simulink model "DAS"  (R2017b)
settings: Solver=FixedStepDiscrete  StartTime=0.0  StopTime=10.0  FixedStep=0.01  RelTol=1e-3  EnableMultiTasking=on
undefined symbols (not defined in the file): CcDAS_ACModeCurtLim_A, CcDAS_ACModeCurtTiLim_ms, CcDAS_BMSOperationConfirmTi_ms, CcDAS_CellMaxTempLim1_C, CcDAS_CellMaxTempLim2_C, CcDAS_CellMaxTempLim3_C, CcDAS_CellMaxTempLim4_C, CcDAS_CellMinTempHiLim_C, CcDAS_CellMinTempLowLim_C, CcDAS_CellMinTempMidLim_C, CcDAS_CellTempDiffLim_C, CcDAS_DCModeCurtTiLim_ms, CcDAS_HVSafetyNVMStoreTi_ms, CcDAS_OCVSOCDiffLim1_numb, CcDAS_OCVSOCDiffLim2_numb, CcDAS_PackCurrLim_A, CcDAS_SOCHighLim_numb, CcDAS_SOCLowerLim_numb, CcDAS_SOHLowerLim_numb, CcDAS_SOHLowerLimSale_numb, DAS_MIN2MS_NUMB, DAS_RUNTIME100_MS, DAS_RUNTIME10_MS, DAS_STATSTIMEMAX_MIN, DAS_STATSTIMEMIN_MIN, DAS_STATSTIMESMAX_NUMB, DAS_STATSTIMESMIN_NUMB, DAS_TIMESONE_NUMB, Enum_CTCCtrCtlConnMode
libraries: AIWAYS_Powertrain_BMS_lib x268
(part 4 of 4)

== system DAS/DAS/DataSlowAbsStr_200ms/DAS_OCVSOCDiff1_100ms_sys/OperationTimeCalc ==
  Enable : EnablePort
  Constant1 : Constant  Value=DAS_MIN2MS_NUMB
  Constant10 : Constant  Value=DAS_RUNTIME100_MS
  Constant2 : Constant  Value=DAS_STATSTIMEMIN_MIN
  Constant3 : Constant  Value=DAS_STATSTIMEMAX_MIN
  Data Store Read : AIWAYS_Powertrain_BMS_lib/Signals/Data Store Read  Priority=0  DSR=EcNVM_OCVSOCDiffTi1_min
  Data Store Write : AIWAYS_Powertrain_BMS_lib/Signals/Data Store Write  DSW=EcNVM_OCVSOCDiffTi1_min
  Data Type Conversion : DataTypeConversion  OutDataTypeStr=single
  Data Type Conversion1 : DataTypeConversion  OutDataTypeStr=single
  Limiter : AIWAYS_Powertrain_BMS_lib/Nonlinear Blocks/Limiter
  OverWrite : AIWAYS_Powertrain_BMS_lib/Signals/OverWrite  OverWrite_Value=CcDAS_OCVSOCDiffTi1Ovr_min  OverWrite_flag=CbDAS_OCVSOCDiffTi1OvrSwt_flg
  Product1 : Product  Inputs=*/  OutDataTypeStr=Inherit: Inherit via back propagation
  Sum : Sum  OutDataTypeStr=Inherit: Inherit via back propagation  RndMeth=Zero
  GcDAS_OCVSOCDiffTi1_min : Outport
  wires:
  Data Store Read/1 -> Sum/1
  Constant10/1 -> Data Type Conversion/1
  Data Type Conversion/1 -> Product1/1
  Product1/1 -> Sum/2
  Constant1/1 -> Data Type Conversion1/1
  Data Type Conversion1/1 -> Product1/2
  Sum/1 -> Limiter/3
  Limiter/1 -> OverWrite/1
  Constant2/1 -> Limiter/2
  Constant3/1 -> Limiter/1
  OverWrite/1 -> Data Store Write/1, GcDAS_OCVSOCDiffTi1_min/1  "GcDAS_OCVSOCDiffTi1_min"

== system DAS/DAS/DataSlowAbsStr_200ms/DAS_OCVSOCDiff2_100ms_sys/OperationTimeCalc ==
  Enable : EnablePort
  Constant1 : Constant  Value=DAS_MIN2MS_NUMB
  Constant10 : Constant  Value=DAS_RUNTIME100_MS
  Constant2 : Constant  Value=DAS_STATSTIMEMIN_MIN
  Constant3 : Constant  Value=DAS_STATSTIMEMAX_MIN
  Data Store Read : AIWAYS_Powertrain_BMS_lib/Signals/Data Store Read  Priority=0  DSR=EcNVM_OCVSOCDiffTi2_min
  Data Store Write : AIWAYS_Powertrain_BMS_lib/Signals/Data Store Write  DSW=EcNVM_OCVSOCDiffTi2_min
  Data Type Conversion : DataTypeConversion  OutDataTypeStr=single
  Data Type Conversion1 : DataTypeConversion  OutDataTypeStr=single
  Limiter : AIWAYS_Powertrain_BMS_lib/Nonlinear Blocks/Limiter
  OverWrite : AIWAYS_Powertrain_BMS_lib/Signals/OverWrite  OverWrite_Value=CcDAS_OCVSOCDiffTi2Ovr_min  OverWrite_flag=CbDAS_OCVSOCDiffTi2OvrSwt_flg
  Product1 : Product  Inputs=*/  OutDataTypeStr=Inherit: Inherit via back propagation
  Sum : Sum  OutDataTypeStr=Inherit: Inherit via back propagation  RndMeth=Zero
  GcDAS_OCVSOCDiffTi2_min : Outport
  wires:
  Data Store Read/1 -> Sum/1
  Constant10/1 -> Data Type Conversion/1
  Data Type Conversion/1 -> Product1/1
  Product1/1 -> Sum/2
  Constant1/1 -> Data Type Conversion1/1
  Data Type Conversion1/1 -> Product1/2
  Sum/1 -> Limiter/3
  Limiter/1 -> OverWrite/1
  Constant2/1 -> Limiter/2
  Constant3/1 -> Limiter/1
  OverWrite/1 -> Data Store Write/1, GcDAS_OCVSOCDiffTi2_min/1  "GcDAS_OCVSOCDiffTi2_min"

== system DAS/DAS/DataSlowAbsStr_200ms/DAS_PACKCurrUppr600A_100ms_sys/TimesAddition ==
  Enable : EnablePort
  ACC_GbACC_ACChrgMismatch_flg : AIWAYS_Powertrain_BMS_lib/Signals/OverWrite  OverWrite_Value=CcDAS_TFPackCrntSafCntOvr_numb  OverWrite_flag=CbDAS_TFPackCrntSafCntOvrSwt_flg
  Constant : Constant  Value=DAS_TIMESONE_NUMB
  Constant4 : Constant  Value=DAS_STATSTIMESMIN_NUMB
  Constant5 : Constant  Value=DAS_STATSTIMESMAX_NUMB
  Data Store Read : AIWAYS_Powertrain_BMS_lib/Signals/Data Store Read  Priority=0  DSR=EcNVM_TFPackCrntSafCnt_numb
  Data Store Write : AIWAYS_Powertrain_BMS_lib/Signals/Data Store Write  DSW=EcNVM_TFPackCrntSafCnt_numb
  Limiter : AIWAYS_Powertrain_BMS_lib/Nonlinear Blocks/Limiter
  Sum : Sum  OutDataTypeStr=Inherit: Inherit via back propagation  RndMeth=Zero
  GcDAS_TFPackCrntSafCnt_numb : Outport
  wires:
  Data Store Read/1 -> Sum/1
  Sum/1 -> Limiter/3
  ACC_GbACC_ACChrgMismatch_flg/1 -> GcDAS_TFPackCrntSafCnt_numb/1, Data Store Write/1  "GcDAS_TFPackCrntSafCnt_numb"
  Constant/1 -> Sum/2
  Constant5/1 -> Limiter/1
  Constant4/1 -> Limiter/2
  Limiter/1 -> ACC_GbACC_ACChrgMismatch_flg/1

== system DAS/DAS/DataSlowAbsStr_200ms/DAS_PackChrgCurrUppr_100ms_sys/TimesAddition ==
  Enable : EnablePort
  ACC_GbACC_ACChrgMismatch_flg : AIWAYS_Powertrain_BMS_lib/Signals/OverWrite  OverWrite_Value=CcDAS_PackChrgCurrUpprLimCntOvr_numb  OverWrite_flag=CbDAS_PackChrgCurrUpprLimCntOvrSwt_flg
  Constant : Constant  Value=DAS_TIMESONE_NUMB
  Constant4 : Constant  Value=DAS_STATSTIMESMIN_NUMB
  Constant5 : Constant  Value=DAS_STATSTIMESMAX_NUMB
  Data Store Read : AIWAYS_Powertrain_BMS_lib/Signals/Data Store Read  Priority=0  DSR=EcNVM_PackChrgCurrUpprLimCnt_numb
  Data Store Write : AIWAYS_Powertrain_BMS_lib/Signals/Data Store Write  DSW=EcNVM_PackChrgCurrUpprLimCnt_numb
  Limiter : AIWAYS_Powertrain_BMS_lib/Nonlinear Blocks/Limiter
  Sum : Sum  OutDataTypeStr=Inherit: Inherit via back propagation  RndMeth=Zero
  GcDAS_PackChrgCurrUpprLimCnt_numb : Outport
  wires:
  Data Store Read/1 -> Sum/1
  Sum/1 -> Limiter/3
  ACC_GbACC_ACChrgMismatch_flg/1 -> GcDAS_PackChrgCurrUpprLimCnt_numb/1, Data Store Write/1  "GcDAS_PackChrgCurrUpprLimCnt_numb"
  Constant/1 -> Sum/2
  Constant5/1 -> Limiter/1
  Constant4/1 -> Limiter/2
  Limiter/1 -> ACC_GbACC_ACChrgMismatch_flg/1

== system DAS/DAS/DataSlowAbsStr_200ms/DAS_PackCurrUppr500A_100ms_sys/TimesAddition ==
  Enable : EnablePort
  ACC_GbACC_ACChrgMismatch_flg : AIWAYS_Powertrain_BMS_lib/Signals/OverWrite  OverWrite_Value=CcDAS_PackCurrLim500ACntOvr_numb  OverWrite_flag=CbDAS_PackCurrLim500ACntOvrSwt_flg
  Constant : Constant  Value=DAS_TIMESONE_NUMB  OutDataTypeStr=single
  Constant4 : Constant  Value=DAS_STATSTIMEMIN_MIN  OutDataTypeStr=single
  Constant5 : Constant  Value=DAS_STATSTIMEMAX_MIN  OutDataTypeStr=single
  Data Store Read : AIWAYS_Powertrain_BMS_lib/Signals/Data Store Read  Priority=0  DSR=EcNVM_PackCurrLim500ACnt_numb
  Data Store Write : AIWAYS_Powertrain_BMS_lib/Signals/Data Store Write  DSW=EcNVM_PackCurrLim500ACnt_numb
  Data Type Conversion : DataTypeConversion  OutDataTypeStr=uint32
  Data Type Conversion1 : DataTypeConversion  OutDataTypeStr=uint32
  Data Type Conversion2 : DataTypeConversion  OutDataTypeStr=uint32
  Limiter : AIWAYS_Powertrain_BMS_lib/Nonlinear Blocks/Limiter
  Sum : Sum  OutDataTypeStr=Inherit: Inherit via back propagation  RndMeth=Zero
  GcDAS_PackCurrLim500ACnt_numb : Outport
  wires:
  Data Store Read/1 -> Sum/1
  Sum/1 -> Limiter/3
  ACC_GbACC_ACChrgMismatch_flg/1 -> GcDAS_PackCurrLim500ACnt_numb/1, Data Store Write/1  "GcDAS_PackCurrLim500ACnt_numb"
  Constant/1 -> Data Type Conversion/1
  Constant5/1 -> Data Type Conversion2/1
  Constant4/1 -> Data Type Conversion1/1
  Limiter/1 -> ACC_GbACC_ACChrgMismatch_flg/1
  Data Type Conversion/1 -> Sum/2
  Data Type Conversion1/1 -> Limiter/2
  Data Type Conversion2/1 -> Limiter/1

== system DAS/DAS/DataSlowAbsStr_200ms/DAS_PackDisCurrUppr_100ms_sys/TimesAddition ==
  Enable : EnablePort
  ACC_GbACC_ACChrgMismatch_flg : AIWAYS_Powertrain_BMS_lib/Signals/OverWrite  OverWrite_Value=CcDAS_PackDisCurrUpprLimCntOvr_numb  OverWrite_flag=CbDAS_PackDisCurrUpprLimCntOvrSwt_flg
  Constant : Constant  Value=DAS_TIMESONE_NUMB
  Constant4 : Constant  Value=DAS_STATSTIMESMIN_NUMB
  Constant5 : Constant  Value=DAS_STATSTIMESMAX_NUMB
  Data Store Read : AIWAYS_Powertrain_BMS_lib/Signals/Data Store Read  Priority=0  DSR=EcNVM_PackDisCurrUpprLimCnt_numb
  Data Store Write : AIWAYS_Powertrain_BMS_lib/Signals/Data Store Write  DSW=EcNVM_PackDisCurrUpprLimCnt_numb
  Limiter : AIWAYS_Powertrain_BMS_lib/Nonlinear Blocks/Limiter
  Sum : Sum  OutDataTypeStr=Inherit: Inherit via back propagation  RndMeth=Zero
  GcDAS_PackDisCurrUpprLimCnt_numb : Outport
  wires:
  Data Store Read/1 -> Sum/1
  Sum/1 -> Limiter/3
  ACC_GbACC_ACChrgMismatch_flg/1 -> GcDAS_PackDisCurrUpprLimCnt_numb/1, Data Store Write/1  "GcDAS_PackDisCurrUpprLimCnt_numb"
  Constant/1 -> Sum/2
  Constant5/1 -> Limiter/1
  Constant4/1 -> Limiter/2
  Limiter/1 -> ACC_GbACC_ACChrgMismatch_flg/1

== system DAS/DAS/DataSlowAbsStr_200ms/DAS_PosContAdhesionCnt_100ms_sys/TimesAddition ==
  Enable : EnablePort
  ACC_GbACC_ACChrgMismatch_flg : AIWAYS_Powertrain_BMS_lib/Signals/OverWrite  OverWrite_Value=CcDAS_PosContAdhesionCntOvr_numb  OverWrite_flag=CbDAS_PosContAdhesionCntOvrSwt_flg
  Constant : Constant  Value=DAS_TIMESONE_NUMB
  Constant4 : Constant  Value=DAS_STATSTIMESMIN_NUMB
  Constant5 : Constant  Value=DAS_STATSTIMESMAX_NUMB
  Data Store Read : AIWAYS_Powertrain_BMS_lib/Signals/Data Store Read  Priority=0  DSR=EcNVM_PosContAdhesionCnt_numb
  Data Store Write : AIWAYS_Powertrain_BMS_lib/Signals/Data Store Write  DSW=EcNVM_PosContAdhesionCnt_numb
  Limiter : AIWAYS_Powertrain_BMS_lib/Nonlinear Blocks/Limiter
  Sum : Sum  OutDataTypeStr=Inherit: Inherit via back propagation  RndMeth=Zero
  GcDAS_PosContAdhesionCnt_numb : Outport
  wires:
  Data Store Read/1 -> Sum/1
  Sum/1 -> Limiter/3
  ACC_GbACC_ACChrgMismatch_flg/1 -> GcDAS_PosContAdhesionCnt_numb/1, Data Store Write/1  "GcDAS_PosContAdhesionCnt_numb"
  Constant/1 -> Sum/2
  Constant5/1 -> Limiter/1
  Constant4/1 -> Limiter/2
  Limiter/1 -> ACC_GbACC_ACChrgMismatch_flg/1

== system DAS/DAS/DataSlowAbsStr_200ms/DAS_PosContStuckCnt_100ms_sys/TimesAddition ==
  Enable : EnablePort
  ACC_GbACC_ACChrgMismatch_flg : AIWAYS_Powertrain_BMS_lib/Signals/OverWrite  OverWrite_Value=CcDAS_PosContStuckCntOvr_numb  OverWrite_flag=CbDAS_PosContStuckCntOvrSwt_flg
  Constant : Constant  Value=DAS_TIMESONE_NUMB
  Constant4 : Constant  Value=DAS_STATSTIMESMIN_NUMB
  Constant5 : Constant  Value=DAS_STATSTIMESMAX_NUMB
  Data Store Read : AIWAYS_Powertrain_BMS_lib/Signals/Data Store Read  Priority=0  DSR=EcNVM_PosContStuckCnt_numb
  Data Store Write : AIWAYS_Powertrain_BMS_lib/Signals/Data Store Write  DSW=EcNVM_PosContStuckCnt_numb
  Limiter : AIWAYS_Powertrain_BMS_lib/Nonlinear Blocks/Limiter
  Sum : Sum  OutDataTypeStr=Inherit: Inherit via back propagation  RndMeth=Zero
  GcDAS_PosContStuckCnt_numb : Outport
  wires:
  Data Store Read/1 -> Sum/1
  Sum/1 -> Limiter/3
  ACC_GbACC_ACChrgMismatch_flg/1 -> GcDAS_PosContStuckCnt_numb/1, Data Store Write/1  "GcDAS_PosContStuckCnt_numb"
  Constant/1 -> Sum/2
  Constant5/1 -> Limiter/1
  Constant4/1 -> Limiter/2
  Limiter/1 -> ACC_GbACC_ACChrgMismatch_flg/1

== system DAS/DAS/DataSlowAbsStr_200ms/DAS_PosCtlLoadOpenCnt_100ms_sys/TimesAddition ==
  Enable : EnablePort
  ACC_GbACC_ACChrgMismatch_flg : AIWAYS_Powertrain_BMS_lib/Signals/OverWrite  OverWrite_Value=CcDAS_PosCtlLoadOpenCntOvr_numb  OverWrite_flag=CbDAS_PosCtlLoadOpenCntOvrSwt_flg
  Constant : Constant  Value=DAS_TIMESONE_NUMB
  Constant4 : Constant  Value=DAS_STATSTIMESMIN_NUMB
  Constant5 : Constant  Value=DAS_STATSTIMESMAX_NUMB
  Data Store Read : AIWAYS_Powertrain_BMS_lib/Signals/Data Store Read  Priority=0  DSR=EcNVM_PosCtlLoadOpenCnt_numb
  Data Store Write : AIWAYS_Powertrain_BMS_lib/Signals/Data Store Write  DSW=EcNVM_PosCtlLoadOpenCnt_numb
  Limiter : AIWAYS_Powertrain_BMS_lib/Nonlinear Blocks/Limiter
  Sum : Sum  OutDataTypeStr=Inherit: Inherit via back propagation  RndMeth=Zero
  GcDAS_PosCtlLoadOpenCnt_numb : Outport
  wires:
  Data Store Read/1 -> Sum/1
  Sum/1 -> Limiter/3
  ACC_GbACC_ACChrgMismatch_flg/1 -> GcDAS_PosCtlLoadOpenCnt_numb/1, Data Store Write/1  "GcDAS_PosCtlLoadOpenCnt_numb"
  Constant/1 -> Sum/2
  Constant5/1 -> Limiter/1
  Constant4/1 -> Limiter/2
  Limiter/1 -> ACC_GbACC_ACChrgMismatch_flg/1

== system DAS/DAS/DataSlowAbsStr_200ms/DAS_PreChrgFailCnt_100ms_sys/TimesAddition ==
  Enable : EnablePort
  ACC_GbACC_ACChrgMismatch_flg : AIWAYS_Powertrain_BMS_lib/Signals/OverWrite  OverWrite_Value=CcDAS_PreChrgFailCntOvr_numb  OverWrite_flag=CbDAS_PreChrgFailCntOvrSwt_flg
  Constant : Constant  Value=DAS_TIMESONE_NUMB
  Constant4 : Constant  Value=DAS_STATSTIMESMIN_NUMB
  Constant5 : Constant  Value=DAS_STATSTIMESMAX_NUMB
  Data Store Read : AIWAYS_Powertrain_BMS_lib/Signals/Data Store Read  Priority=0  DSR=EcNVM_PreChrgFailCnt_numb
  Data Store Write : AIWAYS_Powertrain_BMS_lib/Signals/Data Store Write  DSW=EcNVM_PreChrgFailCnt_numb
  Limiter : AIWAYS_Powertrain_BMS_lib/Nonlinear Blocks/Limiter
  Sum : Sum  OutDataTypeStr=Inherit: Inherit via back propagation  RndMeth=Zero
  GcDAS_PreChrgFailCnt_numb : Outport
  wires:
  Data Store Read/1 -> Sum/1
  Sum/1 -> Limiter/3
  ACC_GbACC_ACChrgMismatch_flg/1 -> GcDAS_PreChrgFailCnt_numb/1, Data Store Write/1  "GcDAS_PreChrgFailCnt_numb"
  Constant/1 -> Sum/2
  Constant5/1 -> Limiter/1
  Constant4/1 -> Limiter/2
  Limiter/1 -> ACC_GbACC_ACChrgMismatch_flg/1

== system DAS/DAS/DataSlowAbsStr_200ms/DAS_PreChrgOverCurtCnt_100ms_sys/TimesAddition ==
  Enable : EnablePort
  ACC_GbACC_ACChrgMismatch_flg : AIWAYS_Powertrain_BMS_lib/Signals/OverWrite  OverWrite_Value=CcDAS_PreChrgOvrCurrCntOvr_numb  OverWrite_flag=CbDAS_PreChrgOvrCurrCntOvrSwt_flg
  Constant : Constant  Value=DAS_TIMESONE_NUMB
  Constant4 : Constant  Value=DAS_STATSTIMESMIN_NUMB
  Constant5 : Constant  Value=DAS_STATSTIMESMAX_NUMB
  Data Store Read : AIWAYS_Powertrain_BMS_lib/Signals/Data Store Read  Priority=0  DSR=EcNVM_PreChrgOvrCurrCnt_numb
  Data Store Write : AIWAYS_Powertrain_BMS_lib/Signals/Data Store Write  DSW=EcNVM_PreChrgOvrCurrCnt_numb
  Limiter : AIWAYS_Powertrain_BMS_lib/Nonlinear Blocks/Limiter
  Sum : Sum  OutDataTypeStr=Inherit: Inherit via back propagation  RndMeth=Zero
  GcDAS_PreChrgOvrCurrCnt_numb : Outport
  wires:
  Data Store Read/1 -> Sum/1
  Sum/1 -> Limiter/3
  ACC_GbACC_ACChrgMismatch_flg/1 -> GcDAS_PreChrgOvrCurrCnt_numb/1, Data Store Write/1  "GcDAS_PreChrgOvrCurrCnt_numb"
  Constant/1 -> Sum/2
  Constant5/1 -> Limiter/1
  Constant4/1 -> Limiter/2
  Limiter/1 -> ACC_GbACC_ACChrgMismatch_flg/1

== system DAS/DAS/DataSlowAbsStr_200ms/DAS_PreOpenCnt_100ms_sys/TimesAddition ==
  Enable : EnablePort
  ACC_GbACC_ACChrgMismatch_flg : AIWAYS_Powertrain_BMS_lib/Signals/OverWrite  OverWrite_Value=CcDAS_PreChrgOpenCntOvr_numb  OverWrite_flag=CbDAS_PreChrgOpenCntOvrSwt_flg
  Constant : Constant  Value=DAS_TIMESONE_NUMB
  Constant4 : Constant  Value=DAS_STATSTIMESMIN_NUMB
  Constant5 : Constant  Value=DAS_STATSTIMESMAX_NUMB
  Data Store Read : AIWAYS_Powertrain_BMS_lib/Signals/Data Store Read  Priority=0  DSR=EcNVM_PreChrgOpenCnt_numb
  Data Store Write : AIWAYS_Powertrain_BMS_lib/Signals/Data Store Write  DSW=EcNVM_PreChrgOpenCnt_numb
  Limiter : AIWAYS_Powertrain_BMS_lib/Nonlinear Blocks/Limiter
  Sum : Sum  OutDataTypeStr=Inherit: Inherit via back propagation  RndMeth=Zero
  GcDAS_PreChrgOpenCnt_numb : Outport
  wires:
  Data Store Read/1 -> Sum/1
  Sum/1 -> Limiter/3
  ACC_GbACC_ACChrgMismatch_flg/1 -> GcDAS_PreChrgOpenCnt_numb/1, Data Store Write/1  "GcDAS_PreChrgOpenCnt_numb"
  Constant/1 -> Sum/2
  Constant5/1 -> Limiter/1
  Constant4/1 -> Limiter/2
  Limiter/1 -> ACC_GbACC_ACChrgMismatch_flg/1

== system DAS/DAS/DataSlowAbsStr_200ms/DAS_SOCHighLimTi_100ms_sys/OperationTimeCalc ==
  Enable : EnablePort
  Constant1 : Constant  Value=DAS_MIN2MS_NUMB
  Constant10 : Constant  Value=DAS_RUNTIME100_MS
  Constant2 : Constant  Value=DAS_STATSTIMEMIN_MIN
  Constant3 : Constant  Value=DAS_STATSTIMEMAX_MIN
  Data Store Read : AIWAYS_Powertrain_BMS_lib/Signals/Data Store Read  Priority=0  DSR=EcNVM_SOCHighLimTi_min
  Data Store Write : AIWAYS_Powertrain_BMS_lib/Signals/Data Store Write  DSW=EcNVM_SOCHighLimTi_min
  Data Type Conversion : DataTypeConversion  OutDataTypeStr=single
  Data Type Conversion1 : DataTypeConversion  OutDataTypeStr=single
  Limiter : AIWAYS_Powertrain_BMS_lib/Nonlinear Blocks/Limiter
  OverWrite : AIWAYS_Powertrain_BMS_lib/Signals/OverWrite  OverWrite_Value=CcDAS_SOCHighLimTiOvr_min  OverWrite_flag=CbDAS_SOCHighLimTiOvrSwt_flg
  Product1 : Product  Inputs=*/  OutDataTypeStr=Inherit: Inherit via back propagation
  Sum : Sum  OutDataTypeStr=Inherit: Inherit via back propagation  RndMeth=Zero
  GcDAS_SOCHighLimTi_min : Outport
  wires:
  Data Store Read/1 -> Sum/1
  Constant10/1 -> Data Type Conversion/1
  Data Type Conversion/1 -> Product1/1
  Product1/1 -> Sum/2
  Constant1/1 -> Data Type Conversion1/1
  Data Type Conversion1/1 -> Product1/2
  Sum/1 -> Limiter/3
  Limiter/1 -> OverWrite/1
  Constant2/1 -> Limiter/2
  Constant3/1 -> Limiter/1
  OverWrite/1 -> Data Store Write/1, GcDAS_SOCHighLimTi_min/1  "GcDAS_SOCHighLimTi_min"

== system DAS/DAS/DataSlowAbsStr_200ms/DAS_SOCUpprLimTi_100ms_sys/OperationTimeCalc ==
  Enable : EnablePort
  Constant1 : Constant  Value=DAS_MIN2MS_NUMB
  Constant10 : Constant  Value=DAS_RUNTIME100_MS
  Constant2 : Constant  Value=DAS_STATSTIMEMIN_MIN
  Constant3 : Constant  Value=DAS_STATSTIMEMAX_MIN
  Data Store Read : AIWAYS_Powertrain_BMS_lib/Signals/Data Store Read  Priority=0  DSR=EcNVM_SOCLowLimTi_min
  Data Store Write : AIWAYS_Powertrain_BMS_lib/Signals/Data Store Write  DSW=EcNVM_SOCLowLimTi_min
  Data Type Conversion : DataTypeConversion  OutDataTypeStr=single
  Data Type Conversion1 : DataTypeConversion  OutDataTypeStr=single
  Limiter : AIWAYS_Powertrain_BMS_lib/Nonlinear Blocks/Limiter
  OverWrite : AIWAYS_Powertrain_BMS_lib/Signals/OverWrite  OverWrite_Value=CcDAS_SOCLowLimTiOvr_min  OverWrite_flag=CbDAS_SOCLowLimTiOvrSwt_flg
  Product1 : Product  Inputs=*/  OutDataTypeStr=Inherit: Inherit via back propagation
  Sum : Sum  OutDataTypeStr=Inherit: Inherit via back propagation  RndMeth=Zero
  GcDAS_SOCLowLimTi_min : Outport
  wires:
  Data Store Read/1 -> Sum/1
  Constant10/1 -> Data Type Conversion/1
  Data Type Conversion/1 -> Product1/1
  Product1/1 -> Sum/2
  Constant1/1 -> Data Type Conversion1/1
  Data Type Conversion1/1 -> Product1/2
  Sum/1 -> Limiter/3
  Limiter/1 -> OverWrite/1
  Constant2/1 -> Limiter/2
  Constant3/1 -> Limiter/1
  OverWrite/1 -> Data Store Write/1, GcDAS_SOCLowLimTi_min/1  "GcDAS_SOCLowLimTi_min"

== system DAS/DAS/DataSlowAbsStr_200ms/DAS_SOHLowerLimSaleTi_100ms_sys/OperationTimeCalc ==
  Enable : EnablePort
  Constant1 : Constant  Value=DAS_MIN2MS_NUMB
  Constant10 : Constant  Value=DAS_RUNTIME100_MS
  Constant2 : Constant  Value=DAS_STATSTIMEMIN_MIN
  Constant3 : Constant  Value=DAS_STATSTIMEMAX_MIN
  Data Store Read : AIWAYS_Powertrain_BMS_lib/Signals/Data Store Read  Priority=0  DSR=EcNVM_SOHLowerLimSaleTi_min
  Data Store Write : AIWAYS_Powertrain_BMS_lib/Signals/Data Store Write  DSW=EcNVM_SOHLowerLimSaleTi_min
  Data Type Conversion : DataTypeConversion  OutDataTypeStr=single
  Data Type Conversion1 : DataTypeConversion  OutDataTypeStr=single
  Limiter : AIWAYS_Powertrain_BMS_lib/Nonlinear Blocks/Limiter
  OverWrite : AIWAYS_Powertrain_BMS_lib/Signals/OverWrite  OverWrite_Value=CcDAS_SOHLowerLimSaleTiOvr_min  OverWrite_flag=CbDAS_SOHLowerLimSaleTiOvrSwt_flg
  Product1 : Product  Inputs=*/  OutDataTypeStr=Inherit: Inherit via back propagation
  Sum : Sum  OutDataTypeStr=Inherit: Inherit via back propagation  RndMeth=Zero
  GcDAS_SOHLowerLimSaleTi_min : Outport
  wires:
  Data Store Read/1 -> Sum/1
  Constant10/1 -> Data Type Conversion/1
  Data Type Conversion/1 -> Product1/1
  Product1/1 -> Sum/2
  Constant1/1 -> Data Type Conversion1/1
  Data Type Conversion1/1 -> Product1/2
  Sum/1 -> Limiter/3
  Limiter/1 -> OverWrite/1
  Constant2/1 -> Limiter/2
  Constant3/1 -> Limiter/1
  OverWrite/1 -> Data Store Write/1, GcDAS_SOHLowerLimSaleTi_min/1  "GcDAS_SOHLowerLimSaleTi_min"

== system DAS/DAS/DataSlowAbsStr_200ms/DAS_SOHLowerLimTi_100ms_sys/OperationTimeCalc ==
  Enable : EnablePort
  Constant1 : Constant  Value=DAS_MIN2MS_NUMB
  Constant10 : Constant  Value=DAS_RUNTIME100_MS
  Constant2 : Constant  Value=DAS_STATSTIMEMIN_MIN
  Constant3 : Constant  Value=DAS_STATSTIMEMAX_MIN
  Data Store Read : AIWAYS_Powertrain_BMS_lib/Signals/Data Store Read  Priority=0  DSR=EcNVM_SOHLowerLimTi_min
  Data Store Write : AIWAYS_Powertrain_BMS_lib/Signals/Data Store Write  DSW=EcNVM_SOHLowerLimTi_min
  Data Type Conversion : DataTypeConversion  OutDataTypeStr=single
  Data Type Conversion1 : DataTypeConversion  OutDataTypeStr=single
  Limiter : AIWAYS_Powertrain_BMS_lib/Nonlinear Blocks/Limiter
  OverWrite : AIWAYS_Powertrain_BMS_lib/Signals/OverWrite  OverWrite_Value=CcDAS_SOHLowerLimTiOvr_min  OverWrite_flag=CbDAS_SOHLowerLimTiOvrSwt_flg
  Product1 : Product  Inputs=*/  OutDataTypeStr=Inherit: Inherit via back propagation
  Sum : Sum  OutDataTypeStr=Inherit: Inherit via back propagation  RndMeth=Zero
  GcDAS_SOHLowerLimTi_min : Outport
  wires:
  Data Store Read/1 -> Sum/1
  Constant10/1 -> Data Type Conversion/1
  Data Type Conversion/1 -> Product1/1
  Product1/1 -> Sum/2
  Constant1/1 -> Data Type Conversion1/1
  Data Type Conversion1/1 -> Product1/2
  Sum/1 -> Limiter/3
  Limiter/1 -> OverWrite/1
  Constant2/1 -> Limiter/2
  Constant3/1 -> Limiter/1
  OverWrite/1 -> Data Store Write/1, GcDAS_SOHLowerLimTi_min/1  "GcDAS_SOHLowerLimTi_min"

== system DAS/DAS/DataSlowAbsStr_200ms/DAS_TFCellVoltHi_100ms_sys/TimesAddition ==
  Enable : EnablePort
  ACC_GbACC_ACChrgMismatch_flg : AIWAYS_Powertrain_BMS_lib/Signals/OverWrite  OverWrite_Value=CcDAS_CellVoltUpprLimCntOvr_numb  OverWrite_flag=CbDAS_CellVoltUpprLimCntOvrSwt_flg
  Constant : Constant  Value=DAS_TIMESONE_NUMB
  Constant4 : Constant  Value=DAS_STATSTIMESMIN_NUMB
  Constant5 : Constant  Value=DAS_STATSTIMESMAX_NUMB
  Data Store Read : AIWAYS_Powertrain_BMS_lib/Signals/Data Store Read  Priority=0  DSR=EcNVM_CellVoltUpprLimCnt_numb
  Data Store Write : AIWAYS_Powertrain_BMS_lib/Signals/Data Store Write  DSW=EcNVM_CellVoltUpprLimCnt_numb
  Limiter : AIWAYS_Powertrain_BMS_lib/Nonlinear Blocks/Limiter
  Sum : Sum  OutDataTypeStr=Inherit: Inherit via back propagation  RndMeth=Zero
  GcDAS_CellVoltUpprLimCnt_numb : Outport
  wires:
  Data Store Read/1 -> Sum/1
  Sum/1 -> Limiter/3
  ACC_GbACC_ACChrgMismatch_flg/1 -> GcDAS_CellVoltUpprLimCnt_numb/1, Data Store Write/1  "GcDAS_CellVoltUpprLimCnt_numb"
  Constant/1 -> Sum/2
  Constant5/1 -> Limiter/1
  Constant4/1 -> Limiter/2
  Limiter/1 -> ACC_GbACC_ACChrgMismatch_flg/1

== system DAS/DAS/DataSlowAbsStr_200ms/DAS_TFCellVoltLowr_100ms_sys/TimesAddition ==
  Enable : EnablePort
  ACC_GbACC_ACChrgMismatch_flg : AIWAYS_Powertrain_BMS_lib/Signals/OverWrite  OverWrite_Value=CcDAS_CellVoltLowrLimCntOvr_numb  OverWrite_flag=CbDAS_CellVoltLowrLimCntOvrSwt_flg
  Constant : Constant  Value=DAS_TIMESONE_NUMB
  Constant4 : Constant  Value=DAS_STATSTIMESMIN_NUMB
  Constant5 : Constant  Value=DAS_STATSTIMESMAX_NUMB
  Data Store Read : AIWAYS_Powertrain_BMS_lib/Signals/Data Store Read  Priority=0  DSR=EcNVM_CellVoltLowrLimCnt_numb
  Data Store Write : AIWAYS_Powertrain_BMS_lib/Signals/Data Store Write  DSW=EcNVM_CellVoltLowrLimCnt_numb
  Limiter : AIWAYS_Powertrain_BMS_lib/Nonlinear Blocks/Limiter
  Sum : Sum  OutDataTypeStr=Inherit: Inherit via back propagation  RndMeth=Zero
  GcDAS_CellVoltLowrLimCnt_numb : Outport
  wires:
  Data Store Read/1 -> Sum/1
  Sum/1 -> Limiter/3
  ACC_GbACC_ACChrgMismatch_flg/1 -> GcDAS_CellVoltLowrLimCnt_numb/1, Data Store Write/1  "GcDAS_CellVoltLowrLimCnt_numb"
  Constant/1 -> Sum/2
  Constant5/1 -> Limiter/1
  Constant4/1 -> Limiter/2
  Limiter/1 -> ACC_GbACC_ACChrgMismatch_flg/1

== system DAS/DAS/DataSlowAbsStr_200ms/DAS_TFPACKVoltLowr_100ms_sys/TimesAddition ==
  Enable : EnablePort
  ACC_GbACC_ACChrgMismatch_flg : AIWAYS_Powertrain_BMS_lib/Signals/OverWrite  OverWrite_Value=CcDAS_BattVoltUpprLimCntOvr_numb  OverWrite_flag=CbDAS_BattVoltUpprLimCntOvrSwt_flg
  Constant : Constant  Value=DAS_TIMESONE_NUMB
  Constant4 : Constant  Value=DAS_STATSTIMESMIN_NUMB
  Constant5 : Constant  Value=DAS_STATSTIMESMAX_NUMB
  Data Store Read : AIWAYS_Powertrain_BMS_lib/Signals/Data Store Read  Priority=0  DSR=EcNVM_BattVoltUpprLimCnt_numb
  Data Store Write : AIWAYS_Powertrain_BMS_lib/Signals/Data Store Write  DSW=EcNVM_BattVoltUpprLimCnt_numb
  Limiter : AIWAYS_Powertrain_BMS_lib/Nonlinear Blocks/Limiter
  Sum : Sum  OutDataTypeStr=Inherit: Inherit via back propagation  RndMeth=Zero
  GcDAS_BattVoltUpprLimCnt_numb : Outport
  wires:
  Data Store Read/1 -> Sum/1
  Sum/1 -> Limiter/3
  ACC_GbACC_ACChrgMismatch_flg/1 -> GcDAS_BattVoltUpprLimCnt_numb/1, Data Store Write/1  "GcDAS_BattVoltUpprLimCnt_numb"
  Constant/1 -> Sum/2
  Constant5/1 -> Limiter/1
  Constant4/1 -> Limiter/2
  Limiter/1 -> ACC_GbACC_ACChrgMismatch_flg/1

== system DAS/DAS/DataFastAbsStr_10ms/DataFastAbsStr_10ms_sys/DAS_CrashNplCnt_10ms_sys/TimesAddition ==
  Enable : EnablePort
  ACC_GbACC_ACChrgMismatch_flg : AIWAYS_Powertrain_BMS_lib/Signals/OverWrite  OverWrite_Value=CcDAS_CrashNplCntOvr_numb  OverWrite_flag=CbDAS_CrashNplCntOvrSwt_flg
  Constant : Constant  Value=DAS_TIMESONE_NUMB  OutDataTypeStr=single
  Constant4 : Constant  Value=DAS_STATSTIMESMIN_NUMB
  Constant5 : Constant  Value=DAS_STATSTIMESMAX_NUMB
  Data Store Read : AIWAYS_Powertrain_BMS_lib/Signals/Data Store Read  Priority=0  DSR=EcNVM_CrashNplCnt_numb
  Data Store Write : AIWAYS_Powertrain_BMS_lib/Signals/Data Store Write  DSW=EcNVM_CrashNplCnt_numb
  Limiter : AIWAYS_Powertrain_BMS_lib/Nonlinear Blocks/Limiter
  Sum : Sum  OutDataTypeStr=Inherit: Inherit via back propagation  RndMeth=Zero
  GcDAS_CrashNplCnt_numb : Outport
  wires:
  Data Store Read/1 -> Sum/1
  Sum/1 -> Limiter/3
  ACC_GbACC_ACChrgMismatch_flg/1 -> GcDAS_CrashNplCnt_numb/1, Data Store Write/1  "GcDAS_CrashNplCnt_numb"
  Constant/1 -> Sum/2
  Constant5/1 -> Limiter/1
  Constant4/1 -> Limiter/2
  Limiter/1 -> ACC_GbACC_ACChrgMismatch_flg/1

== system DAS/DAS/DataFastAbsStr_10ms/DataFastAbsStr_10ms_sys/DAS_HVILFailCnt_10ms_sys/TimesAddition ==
  Enable : EnablePort
  ACC_GbACC_ACChrgMismatch_flg : AIWAYS_Powertrain_BMS_lib/Signals/OverWrite  OverWrite_Value=CcDAS_HVILFailCntOvr_numb  OverWrite_flag=CbDAS_HVILFailCntOvrSwt_flg
  Constant : Constant  Value=DAS_TIMESONE_NUMB
  Constant4 : Constant  Value=DAS_STATSTIMESMIN_NUMB
  Constant5 : Constant  Value=DAS_STATSTIMESMAX_NUMB
  Data Store Read : AIWAYS_Powertrain_BMS_lib/Signals/Data Store Read  Priority=0  DSR=EcNVM_HVILFailCnt_numb
  Data Store Write : AIWAYS_Powertrain_BMS_lib/Signals/Data Store Write  DSW=EcNVM_HVILFailCnt_numb
  Limiter : AIWAYS_Powertrain_BMS_lib/Nonlinear Blocks/Limiter
  Sum : Sum  OutDataTypeStr=Inherit: Inherit via back propagation  RndMeth=Zero
  GcDAS_HVILFailCnt_numb : Outport
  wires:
  Data Store Read/1 -> Sum/1
  Sum/1 -> Limiter/3
  ACC_GbACC_ACChrgMismatch_flg/1 -> GcDAS_HVILFailCnt_numb/1, Data Store Write/1  "GcDAS_HVILFailCnt_numb"
  Constant/1 -> Sum/2
  Constant5/1 -> Limiter/1
  Constant4/1 -> Limiter/2
  Limiter/1 -> ACC_GbACC_ACChrgMismatch_flg/1

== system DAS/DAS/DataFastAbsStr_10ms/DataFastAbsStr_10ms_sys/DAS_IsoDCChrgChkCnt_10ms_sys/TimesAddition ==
  Enable : EnablePort
  ACC_GbACC_ACChrgMismatch_flg : AIWAYS_Powertrain_BMS_lib/Signals/OverWrite  OverWrite_Value=CcDAS_IsoDCChrgChkCntOvr_numb  OverWrite_flag=CbDAS_IsoDCChrgChkCntOvrSwt_flg
  Constant : Constant  Value=DAS_TIMESONE_NUMB
  Constant4 : Constant  Value=DAS_STATSTIMESMIN_NUMB
  Constant5 : Constant  Value=DAS_STATSTIMESMAX_NUMB
  Data Store Read : AIWAYS_Powertrain_BMS_lib/Signals/Data Store Read  Priority=0  DSR=EcNVM_IsoDCChrgChkCnt_numb
  Data Store Write : AIWAYS_Powertrain_BMS_lib/Signals/Data Store Write  DSW=EcNVM_IsoDCChrgChkCnt_numb
  Limiter : AIWAYS_Powertrain_BMS_lib/Nonlinear Blocks/Limiter
  Sum : Sum  OutDataTypeStr=Inherit: Inherit via back propagation  RndMeth=Zero
  GcDAS_IsoDCChrgChkCnt_numb : Outport
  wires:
  Data Store Read/1 -> Sum/1
  Sum/1 -> Limiter/3
  ACC_GbACC_ACChrgMismatch_flg/1 -> GcDAS_IsoDCChrgChkCnt_numb/1, Data Store Write/1  "GcDAS_IsoDCChrgChkCnt_numb"
  Constant/1 -> Sum/2
  Constant5/1 -> Limiter/1
  Constant4/1 -> Limiter/2
  Limiter/1 -> ACC_GbACC_ACChrgMismatch_flg/1

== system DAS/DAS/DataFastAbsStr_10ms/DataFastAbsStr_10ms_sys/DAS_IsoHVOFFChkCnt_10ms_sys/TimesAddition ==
  Enable : EnablePort
  ACC_GbACC_ACChrgMismatch_flg : AIWAYS_Powertrain_BMS_lib/Signals/OverWrite  OverWrite_Value=CcDAS_IsoHVOFFChkCntOvr_numb  OverWrite_flag=CbDAS_IsoHVOFFChkCntOvrSwt_flg
  Constant : Constant  Value=DAS_TIMESONE_NUMB
  Constant4 : Constant  Value=DAS_STATSTIMESMIN_NUMB
  Constant5 : Constant  Value=DAS_STATSTIMESMAX_NUMB
  Data Store Read : AIWAYS_Powertrain_BMS_lib/Signals/Data Store Read  Priority=0  DSR=EcNVM_IsoHVOFFChkCnt_numb
  Data Store Write : AIWAYS_Powertrain_BMS_lib/Signals/Data Store Write  DSW=EcNVM_IsoHVOFFChkCnt_numb
  Limiter : AIWAYS_Powertrain_BMS_lib/Nonlinear Blocks/Limiter
  Sum : Sum  OutDataTypeStr=Inherit: Inherit via back propagation  RndMeth=Zero
  GcDAS_IsoHVOFFChkCnt_numb : Outport
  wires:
  Data Store Read/1 -> Sum/1
  Sum/1 -> Limiter/3
  ACC_GbACC_ACChrgMismatch_flg/1 -> GcDAS_IsoHVOFFChkCnt_numb/1, Data Store Write/1  "GcDAS_IsoHVOFFChkCnt_numb"
  Constant/1 -> Sum/2
  Constant5/1 -> Limiter/1
  Constant4/1 -> Limiter/2
  Limiter/1 -> ACC_GbACC_ACChrgMismatch_flg/1

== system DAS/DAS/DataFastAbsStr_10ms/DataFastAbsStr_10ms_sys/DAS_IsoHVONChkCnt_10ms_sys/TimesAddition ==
  Enable : EnablePort
  ACC_GbACC_ACChrgMismatch_flg : AIWAYS_Powertrain_BMS_lib/Signals/OverWrite  OverWrite_Value=CcDAS_IsoHVOFFChkCntOvr_numb  OverWrite_flag=CbDAS_IsoHVONChkCntOvrSwt_flg
  Constant : Constant  Value=DAS_TIMESONE_NUMB
  Constant4 : Constant  Value=DAS_STATSTIMESMIN_NUMB
  Constant5 : Constant  Value=DAS_STATSTIMESMAX_NUMB
  Data Store Read : AIWAYS_Powertrain_BMS_lib/Signals/Data Store Read  Priority=0  DSR=EcNVM_IsoHVONChkCnt_numb
  Data Store Write : AIWAYS_Powertrain_BMS_lib/Signals/Data Store Write  DSW=EcNVM_IsoHVONChkCnt_numb
  Limiter : AIWAYS_Powertrain_BMS_lib/Nonlinear Blocks/Limiter
  Sum : Sum  OutDataTypeStr=Inherit: Inherit via back propagation  RndMeth=Zero
  GcDAS_IsoHVONChkCnt_numb : Outport
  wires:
  Data Store Read/1 -> Sum/1
  Sum/1 -> Limiter/3
  ACC_GbACC_ACChrgMismatch_flg/1 -> GcDAS_IsoHVONChkCnt_numb/1, Data Store Write/1  "GcDAS_IsoHVONChkCnt_numb"
  Constant/1 -> Sum/2
  Constant5/1 -> Limiter/1
  Constant4/1 -> Limiter/2
  Limiter/1 -> ACC_GbACC_ACChrgMismatch_flg/1

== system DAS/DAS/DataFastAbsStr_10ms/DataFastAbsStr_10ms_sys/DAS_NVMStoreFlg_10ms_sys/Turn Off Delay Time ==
  note: Turn Off Delay Time
  T : Inport
  u : Inport  Port=2
  dT : Inport  Port=3
  AND : Logic  Operator=OR  OutDataTypeStr=boolean
  Constant Value1 : Constant  Value=0  OutDataTypeStr=Inherit: Inherit via back propagation
  Constant Value2 : Constant  Value=0  OutDataTypeStr=Inherit: Inherit via back propagation
  EdgeFalling1 : Subsystem  Tag=R11-1  TreatAsAtomicUnit=on  mask(EdgeFalling){}
      mask help: The output indicates true if the logical input value changes from true to false. Input1=Value (u).
  Greater Than : RelationalOperator  Operator=>  OutDataTypeStr=boolean
  Minimum : MinMax  Function=max  Inputs=2
  Summation : Sum  Inputs=-+
  Switch : Switch  Criteria=u2 ~= 0  Threshold=1  RndMeth=Zero
  Unit Delay : UnitDelay  SampleTime=-1
  y : Outport
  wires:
  T/1 -> Switch/1
  EdgeFalling1/1(y) -> Switch/2
  Constant Value1/1 -> Minimum/2
  Summation/1 -> Minimum/1
  Constant Value2/1 -> Greater Than/2
  Unit Delay/1 -> Summation/2
  u/1 -> EdgeFalling1/1(u), AND/1
  AND/1 -> y/1
  Greater Than/1 -> AND/2
  Switch/1 -> Greater Than/1, Unit Delay/1
  dT/1 -> Summation/1
  Minimum/1 -> Switch/3

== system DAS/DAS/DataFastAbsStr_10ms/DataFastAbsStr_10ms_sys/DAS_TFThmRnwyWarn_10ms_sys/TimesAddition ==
  Enable : EnablePort
  ACC_GbACC_ACChrgMismatch_flg : AIWAYS_Powertrain_BMS_lib/Signals/OverWrite  OverWrite_Value=CcDAS_ThmRnwyWarnCntOvr_numb  OverWrite_flag=CbDAS_ThmRnwyWarnCntOvrSwt_flg
  Constant : Constant  Value=DAS_TIMESONE_NUMB
  Constant4 : Constant  Value=DAS_STATSTIMESMIN_NUMB
  Constant5 : Constant  Value=DAS_STATSTIMESMAX_NUMB
  Data Store Read : AIWAYS_Powertrain_BMS_lib/Signals/Data Store Read  Priority=0  DSR=EcNVM_ThmRnwyWarnCnt_numb
  Data Store Write : AIWAYS_Powertrain_BMS_lib/Signals/Data Store Write  DSW=EcNVM_ThmRnwyWarnCnt_numb
  Limiter : AIWAYS_Powertrain_BMS_lib/Nonlinear Blocks/Limiter
  Sum : Sum  OutDataTypeStr=Inherit: Inherit via back propagation  RndMeth=Zero
  GcDAS_ThmRnwyWarnCnt_numb : Outport
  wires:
  Data Store Read/1 -> Sum/1
  Sum/1 -> Limiter/3
  ACC_GbACC_ACChrgMismatch_flg/1 -> GcDAS_ThmRnwyWarnCnt_numb/1, Data Store Write/1  "GcDAS_ThmRnwyWarnCnt_numb"
  Constant/1 -> Sum/2
  Constant5/1 -> Limiter/1
  Constant4/1 -> Limiter/2
  Limiter/1 -> ACC_GbACC_ACChrgMismatch_flg/1

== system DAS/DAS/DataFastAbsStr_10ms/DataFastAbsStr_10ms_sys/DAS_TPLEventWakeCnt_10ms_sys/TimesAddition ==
  Enable : EnablePort
  ACC_GbACC_ACChrgMismatch_flg : AIWAYS_Powertrain_BMS_lib/Signals/OverWrite  OverWrite_Value=CcDAS_TPLEventWakeCntOvr_numb  OverWrite_flag=CbDAS_TPLEventWakeCntOvrSwt_flg
  Constant : Constant  Value=DAS_TIMESONE_NUMB
  Constant4 : Constant  Value=DAS_STATSTIMESMIN_NUMB
  Constant5 : Constant  Value=DAS_STATSTIMESMAX_NUMB
  Data Store Read : AIWAYS_Powertrain_BMS_lib/Signals/Data Store Read  Priority=0  DSR=EcNVM_TPLEventWakeCnt_numb
  Data Store Write : AIWAYS_Powertrain_BMS_lib/Signals/Data Store Write  DSW=EcNVM_TPLEventWakeCnt_numb
  Limiter : AIWAYS_Powertrain_BMS_lib/Nonlinear Blocks/Limiter
  Sum : Sum  OutDataTypeStr=Inherit: Inherit via back propagation  RndMeth=Zero
  GcDAS_TPLEventWakeCnt_numb : Outport
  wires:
  Data Store Read/1 -> Sum/1
  Sum/1 -> Limiter/3
  ACC_GbACC_ACChrgMismatch_flg/1 -> GcDAS_TPLEventWakeCnt_numb/1, Data Store Write/1  "GcDAS_TPLEventWakeCnt_numb"
  Constant/1 -> Sum/2
  Constant5/1 -> Limiter/1
  Constant4/1 -> Limiter/2
  Limiter/1 -> ACC_GbACC_ACChrgMismatch_flg/1

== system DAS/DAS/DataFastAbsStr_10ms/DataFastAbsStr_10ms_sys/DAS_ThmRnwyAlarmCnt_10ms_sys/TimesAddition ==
  Enable : EnablePort
  ACC_GbACC_ACChrgMismatch_flg : AIWAYS_Powertrain_BMS_lib/Signals/OverWrite  OverWrite_Value=CcDAS_ThmRnwyAlarmCntOvr_numb  OverWrite_flag=CbDAS_ThmRnwyAlarmCntOvrSwt_flg
  Constant : Constant  Value=DAS_TIMESONE_NUMB
  Constant4 : Constant  Value=DAS_STATSTIMESMIN_NUMB
  Constant5 : Constant  Value=DAS_STATSTIMESMAX_NUMB
  Data Store Read : AIWAYS_Powertrain_BMS_lib/Signals/Data Store Read  Priority=0  DSR=EcNVM_ThmRnwyAlarmCnt_numb
  Data Store Write : AIWAYS_Powertrain_BMS_lib/Signals/Data Store Write  DSW=EcNVM_ThmRnwyAlarmCnt_numb
  Limiter : AIWAYS_Powertrain_BMS_lib/Nonlinear Blocks/Limiter
  Sum : Sum  OutDataTypeStr=Inherit: Inherit via back propagation  RndMeth=Zero
  GcDAS_ThmRnwyAlarmCnt_numb : Outport
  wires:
  Data Store Read/1 -> Sum/1
  Sum/1 -> Limiter/3
  ACC_GbACC_ACChrgMismatch_flg/1 -> GcDAS_ThmRnwyAlarmCnt_numb/1, Data Store Write/1  "GcDAS_ThmRnwyAlarmCnt_numb"
  Constant/1 -> Sum/2
  Constant5/1 -> Limiter/1
  Constant4/1 -> Limiter/2
  Limiter/1 -> ACC_GbACC_ACChrgMismatch_flg/1

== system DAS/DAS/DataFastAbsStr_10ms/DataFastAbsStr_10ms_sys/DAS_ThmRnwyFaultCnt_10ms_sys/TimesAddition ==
  Enable : EnablePort
  ACC_GbACC_ACChrgMismatch_flg : AIWAYS_Powertrain_BMS_lib/Signals/OverWrite  OverWrite_Value=CcDAS_ThmRnwyFaultCntOvr_numb  OverWrite_flag=CbDAS_ThmRnwyFaultCntOvrSwt_flg
  Constant : Constant  Value=DAS_TIMESONE_NUMB  OutDataTypeStr=uint16
  Constant4 : Constant  Value=DAS_STATSTIMESMIN_NUMB
  Constant5 : Constant  Value=DAS_STATSTIMESMAX_NUMB
  Data Store Read : AIWAYS_Powertrain_BMS_lib/Signals/Data Store Read  Priority=0  DSR=EcNVM_ThmRnwyFaultCnt_numb
  Data Store Write : AIWAYS_Powertrain_BMS_lib/Signals/Data Store Write  DSW=EcNVM_ThmRnwyFaultCnt_numb
  Limiter : AIWAYS_Powertrain_BMS_lib/Nonlinear Blocks/Limiter
  Sum : Sum  OutDataTypeStr=Inherit: Inherit via back propagation  RndMeth=Zero
  GcDAS_ThmRnwyFaultCnt_numb : Outport
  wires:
  Data Store Read/1 -> Sum/1
  Sum/1 -> Limiter/3
  ACC_GbACC_ACChrgMismatch_flg/1 -> GcDAS_ThmRnwyFaultCnt_numb/1, Data Store Write/1  "GcDAS_ThmRnwyFaultCnt_numb"
  Constant/1 -> Sum/2
  Constant5/1 -> Limiter/1
  Constant4/1 -> Limiter/2
  Limiter/1 -> ACC_GbACC_ACChrgMismatch_flg/1

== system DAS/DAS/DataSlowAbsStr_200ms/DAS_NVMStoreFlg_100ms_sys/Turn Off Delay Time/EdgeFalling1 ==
  note: Edge Falling
  u : Inport  OutDataTypeStr=boolean
  AND : Logic  OutDataTypeStr=boolean
  OR1 : Logic  Operator=NOT  OutDataTypeStr=boolean
  Unit Delay : UnitDelay  SampleTime=-1
  y : Outport  OutDataTypeStr=boolean
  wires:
  u/1 -> Unit Delay/1, OR1/1
  AND/1 -> y/1
  Unit Delay/1 -> AND/2
  OR1/1 -> AND/1

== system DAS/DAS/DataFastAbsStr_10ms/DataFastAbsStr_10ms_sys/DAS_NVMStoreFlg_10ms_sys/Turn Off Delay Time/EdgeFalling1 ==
  note: Edge Falling
  u : Inport  OutDataTypeStr=boolean
  AND : Logic  OutDataTypeStr=boolean
  OR1 : Logic  Operator=NOT  OutDataTypeStr=boolean
  Unit Delay : UnitDelay  SampleTime=-1
  y : Outport  OutDataTypeStr=boolean
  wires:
  u/1 -> Unit Delay/1, OR1/1
  AND/1 -> y/1
  Unit Delay/1 -> AND/2
  OR1/1 -> AND/1
